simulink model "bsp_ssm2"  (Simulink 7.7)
settings: Solver=ode45  StartTime=0.0  StopTime=10  FixedStep=0.1  RelTol=1e-3
libraries: simulink x2

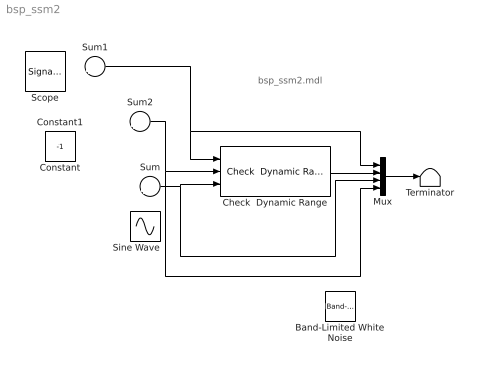
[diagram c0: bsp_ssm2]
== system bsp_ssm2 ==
  note: bsp_ssm2.mdl
  Check  Dynamic Range : simulink/Model Verification/Check  Dynamic Range  Description=min < sig < max  SystemSampleTime=-1  enabled=on  stopWhenAssertionFail=off  export=on  icon=graphic
  Mux : Mux
  Sum : Sum  Inputs=|++
  Sum1 : Sum  Inputs=|++
  Sum2 : Sum  Inputs=|++
  Terminator : Terminator
  Band-Limited White Noise : simulink/Sources/Band-Limited White Noise  IOType=siggen  SystemSampleTime=-1  Cov=[0.001]  Ts=0.01  seed=[23341]
  Constant : Constant  IOType=siggen
  Constant1 : Constant  IOType=siggen  Value=-1
  Scope : SignalViewerScope  IOType=viewer  RefreshTime=0.035000
  Sine Wave : Sin  IOType=siggen  SampleTime=0
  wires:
  Sum1/1 -> Check  Dynamic Range/1, Mux/1
  Mux/1 -> Terminator/1
  Sum/1 -> Check  Dynamic Range/3, Mux/3
  Sum2/1 -> Check  Dynamic Range/2, Mux/4
  Check  Dynamic Range/1 -> Mux/2
